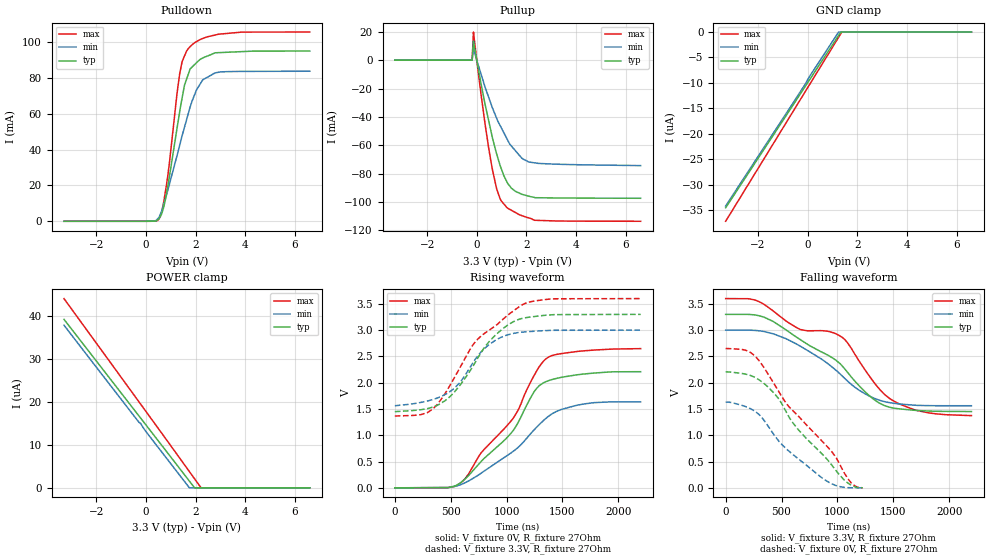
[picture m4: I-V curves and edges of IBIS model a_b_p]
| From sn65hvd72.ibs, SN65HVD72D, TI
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|   a_b Model
[Model]   a_b_p
Model_type   I/O
Polarity   Non-Inverting
Enable   Active-High
Vinl = 0.8
Vinh = 2.0
Vmeas = 1.65
Vref = 1.65
Cref = 50pF
Rref = 27
|   typ   min   max
|   (nom PVT)   (fast PVT)   (slow PVT)
C_comp   1.121e-11   1.058e-11   1.158e-11
|ON state : BUFFER OUTPUT TURNED HIGH
|C_comp   1.312e-11   1.240e-11   1.351e-11
|OFF state: BUFFER IN HIGH IMPEDANCE
|C_comp   9.313e-12   8.774e-12   9.661e-12
| Where nom  PVT is Nominal Process, 3.3V, 27C
|   Fast PVT is Strong Process,  3.6V, -40C
|   Slow PVT is Weak Process,   3V, 125C
[Voltage Range]   3.3   3   3.6
[Temperature Range]   27   125   -40
[Pullup Reference]   3.3   3   3.6
[Pulldown Reference]   0   0   0
[Power Clamp Reference]   3.3   3   3.6
[GND Clamp Reference]   0   0   0
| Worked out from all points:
|   slope of the pulldown table from 0 to 0.495 V, typ, clamps not added: 498 ohm
|   slope of the pullup table from 0 to 0.495 V, typ, clamps not added: 11.3 ohm
|   falling waveform, V_fixture 3.3V, R_fixture 27Ohm: 20-80 % time 660ns typ, 547ns min, 849ns max; typ from 3.3 V to 1.45 V
|   rising waveform, V_fixture 0V, R_fixture 27Ohm: 20-80 % time 483ns typ, 539ns min, 510ns max; typ from 0 V to 2.21 V
|   rising waveform, V_fixture 3.3V, R_fixture 27Ohm: 20-80 % time 381ns typ, 332ns min, 485ns max; typ from 1.45 V to 3.3 V
|   falling waveform, V_fixture 0V, R_fixture 27Ohm: 20-80 % time 499ns typ, 446ns min, 607ns max; typ from 2.2 V to 0.001 V
[Pulldown]
|   Voltage   I(typ)   I(min)   I(max)
-3.3V     -1.604nA   -10.59nA   0A
478.8mV   854.1uA    1.46mA     485.5uA
633.6mV   4.157mA    5.701mA    5.209mA
828mV     15.47mA    14.57mA    20.22mA
1.278V    54.06mA    37.94mA    74.06mA
1.451V    68.27mA    47.35mA    88.61mA
1.554V    75.96mA    52.52mA    92.24mA
1.782V    85.03mA    63.83mA    97.48mA
1.922V    86.9mA     69.27mA    99.2mA
2.283V    91.04mA    78.8mA     102mA
2.781V    93.97mA    82.73mA    103.9mA
6.6V      94.94mA    83.7mA     105.6mA
[GND Clamp]
|   Voltage   I(typ)   I(min)   I(max)
-3.3V     -34.52uA   -34.17uA   -37.17uA
-579mV    -14.29uA   -13.88uA   -15.55uA
-117mV    -10.85uA   -10.4uA    -11.88uA
93mV      -9.28uA    -8.621uA   -10.21uA
1.248V    -686.6nA   -1.892nA   -1.032uA
1.34V     -2.32nA    0A         -300.4nA
1.375V    0A         0A         -18.23nA
6.6V      0A         0A         0A
[Pullup]
|   Voltage   I(typ)   I(min)   I(max)
-3.3V     0A         0A         0A
-186mV    0A         0A         0A
-133.2mV  13.33mA    8.265mA    19.81mA
61.2mV    -5.892mA   -3.527mA   -8.761mA
338.4mV   -31.41mA   -19.2mA    -45.44mA
633.6mV   -54.91mA   -33.77mA   -77.41mA
795.6mV   -65.81mA   -40.76mA   -90.26mA
939.6mV   -74.23mA   -46.06mA   -97.67mA
1.21V     -85.62mA   -55.2mA    -103.9mA
1.554V    -92.43mA   -63.79mA   -107.4mA
2.091V    -95.87mA   -71.78mA   -111.2mA
6.6V      -97.38mA   -74.35mA   -113.6mA
[POWER Clamp]
|   Voltage   I(typ)   I(min)   I(max)
-3.3V     39.17uA    37.81uA    43.99uA
-309mV    16.92uA    15.45uA    20.22uA
-213mV    16.21uA    15.01uA    19.46uA
18mV      14.49uA    12.96uA    17.62uA
1.749V    1.573uA    20.51nA    3.787uA
1.957V    22.28nA    0A         2.122uA
2.221V    0A         0A         10.48nA
6.6V      0A         0A         0A
[Ramp]
R_load = 27
|   typ   min   max
dV/dt_r   1.32551/4.82476e-07   0.980085/5.39764e-07   1.58885/5.09671e-07
dV/dt_f   1.10898/6.61224e-07   0.862702/5.46246e-07   1.33541/8.49121e-07
[Falling Waveform]
V_fixture = 3.3V
V_fixture_min = 3V
V_fixture_max = 3.6V
R_fixture = 27Ohm
|   Time   V(typ)   V(min)   V(max)
0s        3.3V       3V         3.6V
264ns     3.289V     2.995V     3.572V
427.9ns   3.162V     2.929V     3.361V
669.5ns   2.818V     2.693V     3.011V
1.024us   2.363V     2.168V     2.89V
1.092us   2.194V     2.028V     2.756V
1.262us   1.799V     1.772V     2.199V
1.424us   1.563V     1.639V     1.773V
1.72us    1.471V     1.569V     1.468V
2.2us     1.452V     1.562V     1.374V
[Rising Waveform]
|Vcc
V_fixture = 0V
V_fixture_min = 0V
V_fixture_max = 0V
R_fixture = 27Ohm
|   Time   V(typ)   V(min)   V(max)
0s        268.8uV    251.9uV    295.4uV
476.4ns   5.371mV    7.49mV     4.343mV
595.1ns   107.5mV    65.76mV    103.9mV
660.4ns   234.5mV    130.7mV    264.9mV
768.5ns   492.2mV    273.1mV    654.5mV
1.066us   1.109V     704.9mV    1.344V
1.253us   1.845V     1.117V     2.16V
1.379us   2.041V     1.367V     2.491V
1.689us   2.165V     1.595V     2.606V
2.2us     2.209V     1.634V     2.648V
[Rising Waveform]
V_fixture = 3.3V
V_fixture_min = 3V
V_fixture_max = 3.6V
R_fixture = 27Ohm
|   Time   V(typ)   V(min)   V(max)
0s        1.45V      1.562V     1.366V
233.5ns   1.486V     1.625V     1.393V
342.1ns   1.537V     1.681V     1.505V
532.4ns   1.82V      1.894V     2.093V
725.4ns   2.407V     2.462V     2.793V
815.8ns   2.708V     2.675V     2.958V
911.4ns   2.926V     2.821V     3.1V
1.155us   3.23V      2.965V     3.498V
1.429us   3.295V     2.997V     3.596V
2.2us     3.3V       3V         3.6V
[Falling Waveform]
V_fixture = 0V
V_fixture_min = 0V
V_fixture_max = 0V
R_fixture = 27Ohm
|   Time   V(typ)   V(min)   V(max)
0s        2.204V     1.629V     2.649V
174.3ns   2.165V     1.549V     2.621V
272.7ns   2.088V     1.44V      2.484V
432.4ns   1.804V     1.01V      1.983V
545.4ns   1.432V     737.1mV    1.598V
646.1ns   1.117V     559.4mV    1.376V
851.5ns   669mV      206.4mV    913.7mV
986.9ns   330.6mV    43.8mV     579.7mV
1.125us   47.91mV    1.542mV    92.02mV
1.227us   510.2uV    422.2uV    171.6uV
